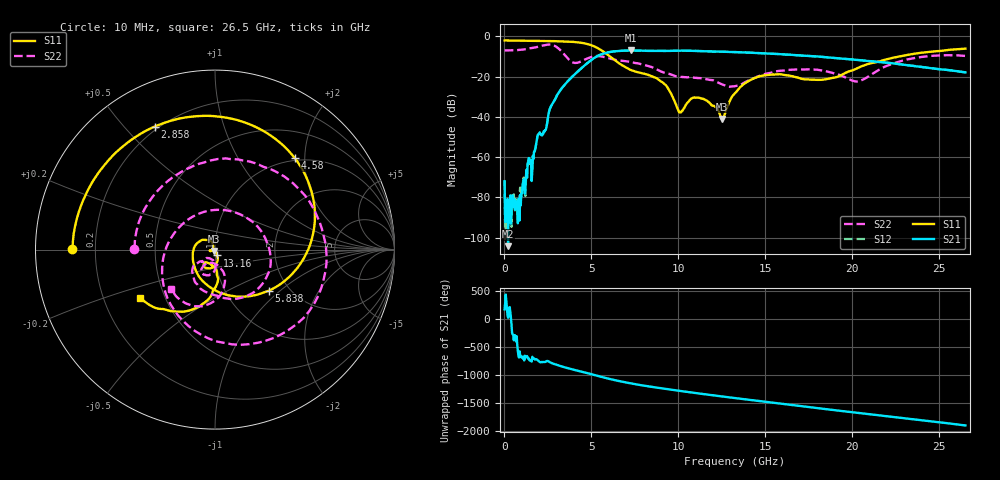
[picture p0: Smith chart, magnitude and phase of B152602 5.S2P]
!  2-Port S-parameters saved by WinCal
! VAR MeasName=S-Parameters (CALIBRATED_DATA) read from VNA (N5242A)
! VAR MeasDate=2016-1-5 16:26:19
! VAR NAME=B152602 5
! VAR FILENAME=B152602 5.S2P
! VAR DATE=2016-1-5 16:26:19
! VAR PHYS_PORTS=1,2
# Hz S DB R 50
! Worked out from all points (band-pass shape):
!   801 points, 10 MHz to 26.5 GHz, reference 50 ohm
!   highest |S21| = -6.97 dB at 7.295 GHz (marker M1); lowest = -104.3 dB at 208.7 MHz (marker M2)
!   |S21| within 3 dB of the highest: 5.31 GHz to 17.99 GHz (12.68 GHz wide, 109 % of centre)
!   lowest |S11| = -41.0 dB at 12.53 GHz (marker M3), VSWR 1.02, Z = 49.5 - j0.748 ohm
!   |S11| at or under -10 dB: 6.075 GHz to 22.68 GHz (16.61 GHz wide, 116 % of centre)
!   |S22| runs from -25.0 to -4.0 dB; largest |S21 - S12| = 0.0024
!   S11 on the Smith chart (normalised r, x): 10 MHz: 0.11, +0.00; 2.858 GHz: 0.18, +0.61; 4.58 GHz: 0.96, +1.80; 5.838 GHz: 1.58, -0.84; 13.16 GHz: 1.02, -0.07; 26.5 GHz: 0.36, -0.26
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1e7  -2.00 179.7  -71.97 178.2  -72.03 -169.2  -6.96 179.4
2.08675e8  -2.02 175.7  -104.31 27.8  -82.55 -135.1  -6.95 167.1
8.70925e8  -2.09 162.1  -91.57 147.6  -78.02 52.8  -6.70 126.0
1.73185e9  -2.20 143.9  -57.25 15.1  -57.18 17.8  -5.50 65.2
2.427212e9  -2.28 127.7  -44.61 -26.6  -44.74 -26.6  -4.17 0.5
2.857675e9  -2.34 116.1  -32.05 -78.8  -32.06 -78.9  -4.55 -56.0
3.519925e9  -2.52 95.5  -23.46 -143.2  -23.47 -143.3  -9.74 -154.8
4.447075e9  -3.20 55.9  -15.59 142.7  -15.60 142.8  -12.27 51.9
4.579525e9  -3.40 48.8  -14.60 132.9  -14.62 132.9  -11.69 36.4
5.8378e9  -8.46 -37.3  -8.15 30.3  -8.13 30.4  -10.43 -65.1
7.29475e9  -16.79 -144.3  -6.97 -67.2  -6.98 -67.2  -12.77 -111.4
8.851038e9  -21.46 139.5  -7.15 -144.9  -7.15 -145.0  -16.81 -143.2
1.00762e10  -37.66 150.9  -7.07 161.4  -7.06 161.3  -19.99 -139.2
1.11358e10  -30.39 -169.9  -7.25 115.9  -7.24 116.0  -20.69 -135.4
1.252652e10  -41.03 -121.8  -7.61 60.5  -7.60 60.4  -23.91 -132.9
1.315566e10  -29.13 -69.9  -7.76 35.8  -7.75 35.7  -24.82 -112.3
1.3255e10  -28.18 -70.8  -7.79 31.9  -7.79 31.8  -24.73 -108.2
1.491062e10  -19.38 -103.7  -8.44 -31.9  -8.39 -32.1  -18.91 -90.5
1.769208e10  -21.51 -118.0  -9.80 -136.4  -9.78 -136.3  -16.39 -116.1
2.027485e10  -15.89 -84.0  -11.71 129.0  -11.65 128.9  -22.42 -99.5
2.209604e10  -11.06 -97.5  -13.18 63.0  -13.11 62.9  -14.29 -73.6
2.65e10  -6.09 -147.2  -17.87 -97.3  -17.85 -97.8  -9.70 -138.4
